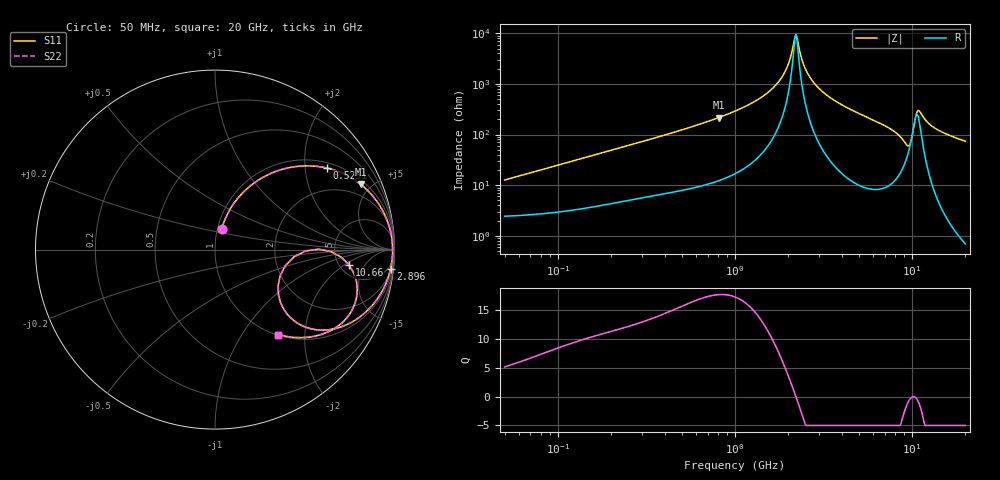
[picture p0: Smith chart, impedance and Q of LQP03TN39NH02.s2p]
!Murata Part Number: LQP03TN39NH02
!These Parameters are Measured in Series Mode Connection
!  o--[Z]--o
!Port1  Port2
!  o-------o
!Freq. Start=50[MHz] Stop=20[GHz], 401[Steps]
# Hz S RI R 50
!Freq.(Hz) S11(Real) S11(Imag) S21(Real) S21(Imag) S12(Real) S12(Imag) S22(Real) S22(Imag)
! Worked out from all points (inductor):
!   401 points, 50 MHz to 20 GHz, reference 50 ohm
!   read as one part in series: L = 39.5 nH near 51.52 MHz
!   highest Q = 17.6 at 810.8 MHz (marker M1), where L = 42.6 nH
!   self-resonance near 2.179 GHz
!   S11 on the Smith chart (normalised r, x): 50 MHz: 1.05, +0.25; 525.1 MHz: 1.16, +2.60; 2.896 GHz: 3, -18; 10.66 GHz: 6.09, -2.35; 20 GHz: 1.01, -1.47
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5e7  0.038 0.1169  0.962 -0.1169  0.962 -0.1169  0.038 0.1169
1.364002e8  0.1251 0.2837  0.8749 -0.2837  0.8749 -0.2837  0.1251 0.2837
3.721004e8  0.4545 0.4634  0.5455 -0.4634  0.5455 -0.4634  0.4545 0.4634
5.251442e8  0.6219 0.4545  0.3781 -0.4545  0.3781 -0.4545  0.6219 0.4545
8.108264e8  0.8117 0.3636  0.1883 -0.3636  0.1883 -0.3636  0.8117 0.3636
1e9  0.8805 0.2966  0.1195 -0.2966  0.1195 -0.2966  0.8805 0.2966
1.369645e9  0.9508 0.1828  0.0492 -0.1828  0.0492 -0.1828  0.9508 0.1828
1.714689e9  0.9785 0.0974  0.0215 -0.0974  0.0215 -0.0974  0.9785 0.0974
1.962148e9  0.987 0.0455  0.013 -0.0455  0.013 -0.0455  0.987 0.0455
2.211938e9  0.9896 -0.000879  0.0104 0.000879  0.0104 0.000879  0.9896 -0.000879
2.456456e9  0.9881 -0.0418  0.0119 0.0418  0.0119 0.0418  0.9881 -0.0418
2.728004e9  0.983 -0.0829  0.017 0.0829  0.017 0.0829  0.983 -0.0829
2.896447e9  0.9784 -0.1066  0.0216 0.1066  0.0216 0.1066  0.9784 -0.1066
4.087748e9  0.9239 -0.2445  0.0761 0.2445  0.0761 0.2445  0.9239 -0.2445
7.442007e9  0.6309 -0.4467  0.3691 0.4467  0.3691 0.4467  0.6309 -0.4467
8.644534e9  0.4487 -0.4027  0.5513 0.4027  0.5513 0.4027  0.4487 -0.4027
9.457416e9  0.3516 -0.2015  0.6484 0.2015  0.6484 0.2015  0.3516 -0.2015
1.004137e10  0.5041 -0.00773  0.4959 0.00773  0.4959 0.00773  0.5041 -0.00773
1.066139e10  0.7458 -0.0842  0.2542 0.0842  0.2542 0.0842  0.7458 -0.0842
1.131968e10  0.7901 -0.2578  0.2099 0.2578  0.2099 0.2578  0.7901 -0.2578
1.295331e10  0.6714 -0.4357  0.3286 0.4357  0.3286 0.4357  0.6714 -0.4357
2e10  0.353 -0.4732  0.647 0.4732  0.647 0.4732  0.353 -0.4732
